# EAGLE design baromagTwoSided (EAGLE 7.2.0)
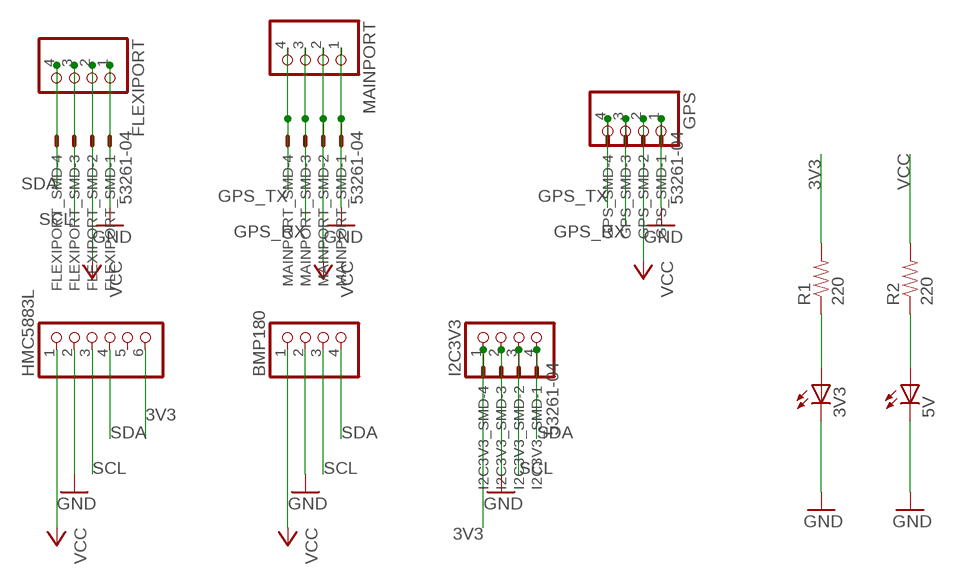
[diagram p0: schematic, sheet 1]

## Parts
3V3  LEDCHIP-LED0805  [CHIP-LED0805]
5V  LEDCHIP-LED0805  [CHIP-LED0805]
BMP180  PINHD-1X4  [1X04]
FLEXIPORT  PINHD-1X4_2.54-SMD-90°  [1X04SMD/90]
FLEXIPORT_SMD  53261-04  [53261-04]
GPS  PINHD-1X4_2.54-SMD-90°  [1X04SMD/90]
GPS_SMD  53261-04  [53261-04]
HMC5883L  PINHD-1X6_2.54  [1X06]
I2C3V3  PINHD-1X4  [1X04]
I2C3V3_SMD  53261-04  [53261-04]
MAINPORT  PINHD-1X4_2.54-SMD-90°  [1X04SMD/90]
MAINPORT_SMD  53261-04  [53261-04]
R1  220  0.22OHM-1/4W-1%(0805)  [0805]
R2  220  0.22OHM-1/4W-1%(0805)  [0805]

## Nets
3V3: HMC5883L.6 I2C3V3.1 I2C3V3_SMD.4 R1.2
GND: 3V3.C 5V.C BMP180.2 FLEXIPORT.1 FLEXIPORT_SMD.1 GPS.1 GPS_SMD.1 HMC5883L.2 I2C3V3.2 I2C3V3_SMD.3 MAINPORT.1 MAINPORT_SMD.1
GPS_RX: GPS.3 GPS_SMD.3 MAINPORT.3 MAINPORT_SMD.3
GPS_TX: GPS.4 GPS_SMD.4 MAINPORT.4 MAINPORT_SMD.4
N$1: 3V3.A R1.1
N$2: 5V.A R2.1
SCL: BMP180.3 FLEXIPORT.3 FLEXIPORT_SMD.3 HMC5883L.3 I2C3V3.3 I2C3V3_SMD.2
SDA: BMP180.4 FLEXIPORT.4 FLEXIPORT_SMD.4 HMC5883L.4 I2C3V3.4 I2C3V3_SMD.1
VCC: BMP180.1 FLEXIPORT.2 FLEXIPORT_SMD.2 GPS.2 GPS_SMD.2 HMC5883L.1 MAINPORT.2 MAINPORT_SMD.2 R2.2
Unconnected: HMC5883L.5

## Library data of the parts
3V3 5V = adafruit:LED: LED
BMP180 I2C3V3 = pinhead:PINHD-1X4: PIN HEADER
FLEXIPORT GPS MAINPORT = pinhead-1:PINHD-1X4: PIN HEADER
FLEXIPORT_SMD GPS_SMD I2C3V3_SMD MAINPORT_SMD = con-molex:53?-04: CONNECTOR wire to board 1.25 mm (.049 inch) pitch header
HMC5883L = pinhead-1:PINHD-1X6: PIN HEADER
R1 R2 = SparkFun-Resistors:0.22OHM-1/4W-1%(0805): RES-09883; PROD_ID: RES-09883; VALUE: 0.22

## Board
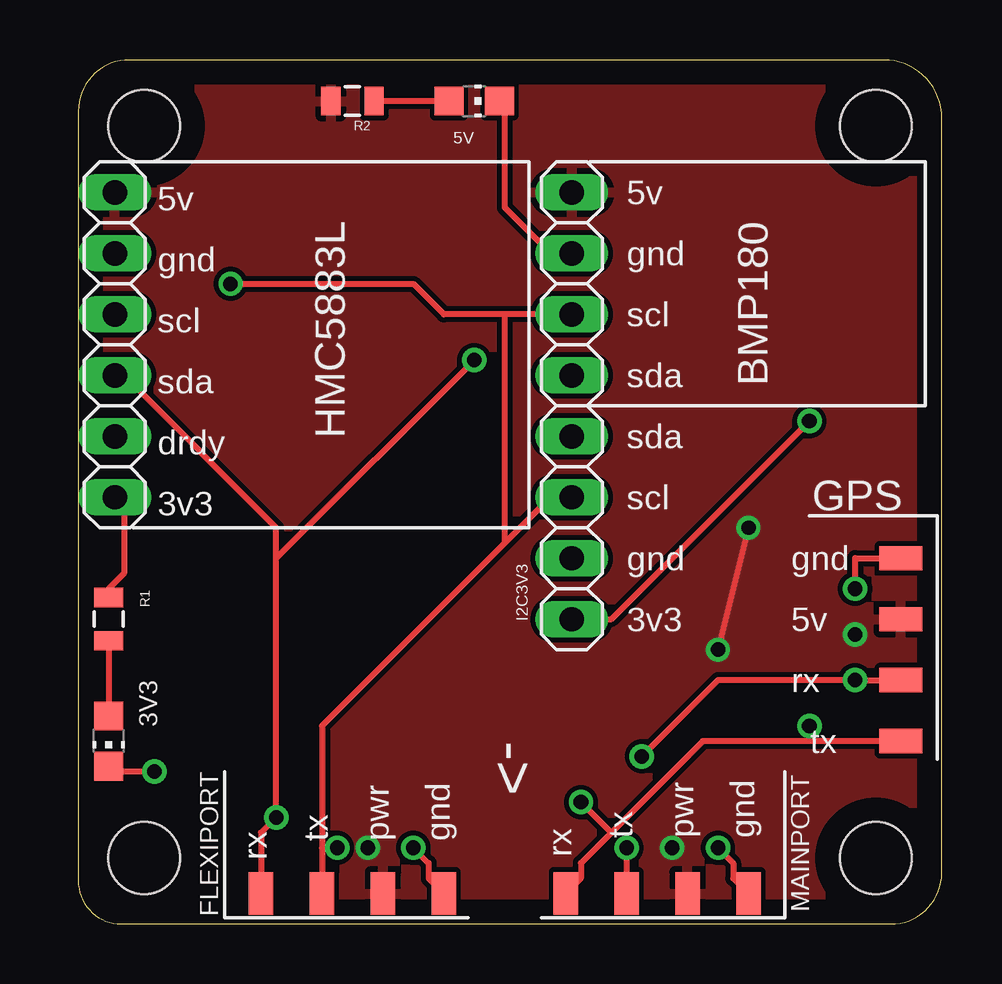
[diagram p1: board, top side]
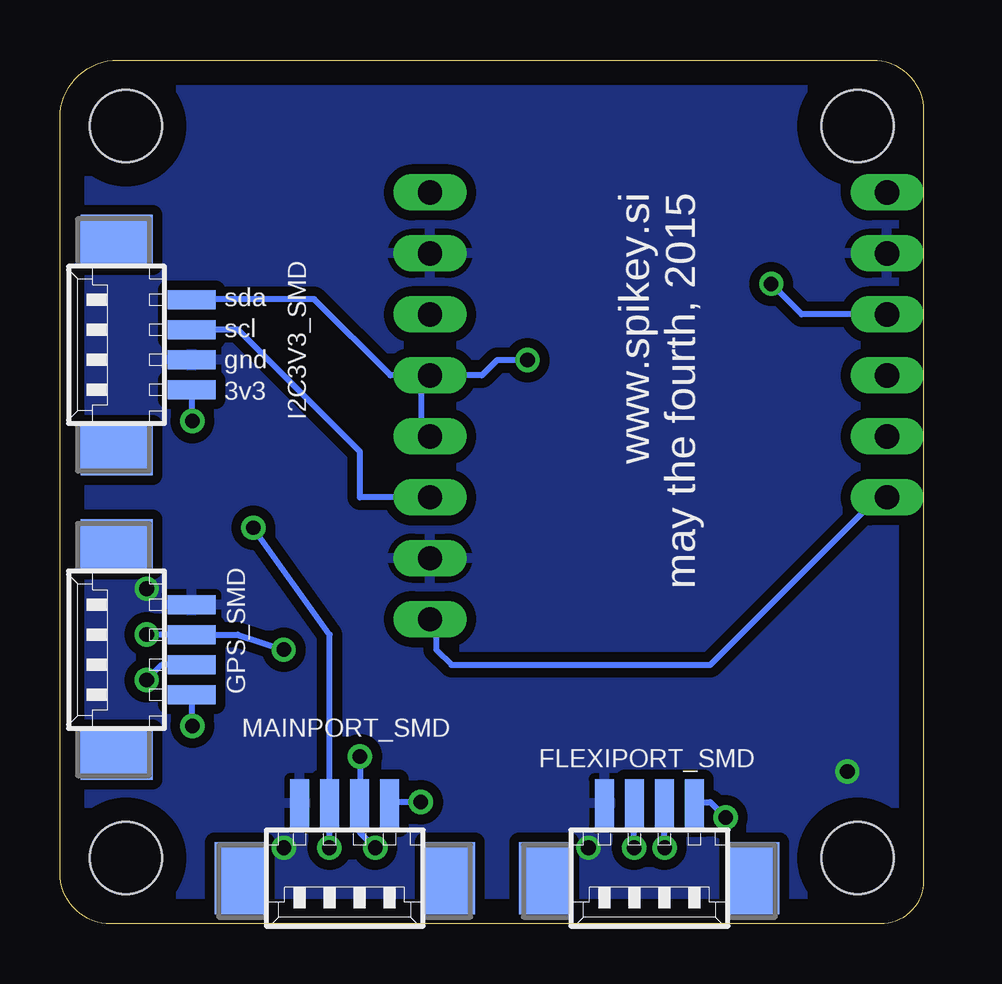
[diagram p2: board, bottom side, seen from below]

Size 36 x 36 mm. Coordinates in mm from the lower left corner, seen from the top.
Outline: 0,33.87 0,1.8 arc90 1.8,0 33.87,0 arc90 36,2.13 36,33.58 arc90 33.58,36 2.13,36 arc90 0,33.87
Copper layers (1*16): Top 0.035mm / dielectric 1.5mm / Bottom 0.035mm
Design rules "default": minimum track width 10mil, minimum drill 24mil, track to track 8mil, track to pad 8mil, pad to pad 8mil, via to via 8mil, smd to smd 8mil, copper to edge 40mil, drill to drill 8mil, minimum pad ring 10mil, minimum via ring 8mil, stop-mask expansion 4mil, vias tented up to drill 0mil, thermal gap 10mil
Holes 3 mm at 2.75,2.75 33.25,2.75 33.25,33.25 2.75,33.25

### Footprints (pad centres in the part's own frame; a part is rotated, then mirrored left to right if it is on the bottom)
CHIP-LED0805 = smd 1.2 x 1.2: A 0,-1.05; C 0,1.05
1X04 = drill 1.016 long: 1 -3.81,0; 2 -1.27,0; 3 1.27,0; 4 3.81,0
1X04SMD/90 = smd 1.016 x 1.778: 1 -1.27,-5.08; 2 1.27,-5.08; 3 3.81,-5.08; 4 6.35,-5.08
53261-04 = smd 0.8 x 2: 1 1.875,-2.5; 2 0.625,-2.5; 3 -0.625,-2.5; 4 -1.875,-2.5 | smd 2.1 x 3: S1 4.375,0.625; S2 -4.375,0.625
1X06 = drill 1.016 long: 1 -6.35,0; 2 -3.81,0; 3 -1.27,0; 4 1.27,0; 5 3.81,0; 6 6.35,0
0805 = smd 0.8 x 1.2: 1 -0.9,0; 2 0.9,0

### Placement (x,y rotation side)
3V3  1.27,7.62 180 top
5V  16.51,34.29 270 top
BMP180  20.57,26.67 270 top
FLEXIPORT  13.97,-3.81 180 top
FLEXIPORT_SMD  11.43,2.54 180 bottom
GPS  39.37,13.97 270 top
GPS_SMD  33.02,11.43 90 bottom
HMC5883L  1.52,24.13 270 top
I2C3V3  20.57,16.51 90 top
I2C3V3_SMD  33.02,24.13 90 bottom
MAINPORT  26.67,-3.81 180 top
MAINPORT_SMD  24.13,2.54 180 bottom
R1  1.27,12.7 90 top
R2  11.43,34.29 180 top

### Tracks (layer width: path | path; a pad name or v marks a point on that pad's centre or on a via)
3V3  (via drill 0.61)
  Top 0.254: R1.2 1.27,13.97 1.91,14.61 1.91,17.78 HMC5883L.6 | v30.48,20.95 22.23,12.7 I2C3V3.1
  Bottom 0.254: v30.48,20.95 30.48,22.23 I2C3V3_SMD.4 | HMC5883L.6 1.91,17.78 8.89,10.79 19.68,10.79 20.32,11.43 20.32,12.7 I2C3V3.1
GND  (via drill 0.61)
  Top 0.254: v3.17,6.35 1.27,6.35 3V3.C | BMP180.2 19.68,27.94 17.78,29.84 17.78,34.29 5V.C | FLEXIPORT.1 14.61,1.91 14.61,2.54 v13.97,3.17 | MAINPORT.1 27.3,1.91 27.3,2.54 v26.67,3.17 | GPS.1 32.38,15.24 v32.38,13.97
  pour Bottom (isolate 0.406): 0,0 38.1,0 38.1,36.83 0,36.83
GPS_RX  (via drill 0.61)
  Top 0.254: v22.86,3.17 MAINPORT.3 | GPS.3 v32.38,10.16 26.67,10.16 v23.5,6.99
  Bottom 0.254: v22.86,3.17 23.5,3.81 23.5,4.45 MAINPORT_SMD.3 23.5,5.08 v23.5,6.99 | v32.38,10.16 31.75,10.79 31.11,10.79 GPS_SMD.3
GPS_TX  (via drill 0.61)
  Top 0.254: MAINPORT.4 20.95,1.91 20.95,2.54 22.23,3.81 | 22.23,3.81 26.04,7.62 30.48,7.62 | GPS.4 30.48,7.62 | 22.23,3.81 v20.95,5.08 | 30.48,7.62 v30.48,8.26
  Bottom 0.254: v20.95,5.08 22.23,5.08 MAINPORT_SMD.4 | v30.48,8.26 30.48,9.53 GPS_SMD.4
N$1
  Top 0.254: R1.1 3V3.A
N$2
  Top 0.254: 5V.A R2.1
SCL  (via drill 0.6, 0.61)
  Top 0.254: BMP180.3 17.78,25.4 | 10.16,3.17 10.16,8.26 17.78,15.88 | 10.16,3.17 FLEXIPORT.3 | I2C3V3.3 19.68,17.78 17.78,15.88 | 10.16,3.17 v10.79,3.17 | 17.78,15.88 17.78,25.4 | 17.78,25.4 15.24,25.4 13.97,26.67 v6.35,26.67
  Bottom 0.254: v10.79,3.17 10.79,4.45 FLEXIPORT_SMD.3 | I2C3V3.3 23.5,17.78 23.5,19.68 28.57,24.77 30.48,24.77 I2C3V3_SMD.2 | HMC5883L.3 5.08,25.4 v6.35,26.67
SDA  (via drill 0.61)
  Top 0.254: FLEXIPORT.4 7.62,3.81 v8.26,4.45 8.26,15.24 | 8.26,15.24 8.26,16.51 1.91,22.86 HMC5883L.4 | 8.26,15.24 v16.51,23.5
  Bottom 0.254: 20.95,22.86 22.23,22.86 25.4,26.04 30.48,26.04 I2C3V3_SMD.1 | 20.95,22.86 20.95,20.32 I2C3V3.4 | 20.95,22.86 BMP180.4 18.41,22.86 17.78,23.5 v16.51,23.5 | v8.26,4.45 8.89,5.08 9.53,5.08 FLEXIPORT_SMD.4
VCC  (via drill 0.6, 0.61)
  Top 0.254: v27.94,16.51 v26.67,11.43
  Bottom 0.254: v12.06,3.17 12.06,4.45 FLEXIPORT_SMD.2 | v24.77,3.17 24.77,4.45 MAINPORT_SMD.2 24.75,12.05 v27.94,16.51 | v32.38,12.06 31.11,12.06 GPS_SMD.2 28.59,12.05 v26.67,11.43
  pour Top: 0,0 36.83,0 36.83,38.1 0,38.1

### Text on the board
tNames: 5v / gnd / scl / sda / drdy / 3v3 | 5v / gnd / scl / sda / sda / scl / gnd / 3v3 | <- | gnd / 5v / rx / tx | rx / tx / pwr / gnd | rx / tx / pwr / gnd
bNames: www.spikey.si / may the fourth, 2015 | sda / scl / gnd / 3v3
